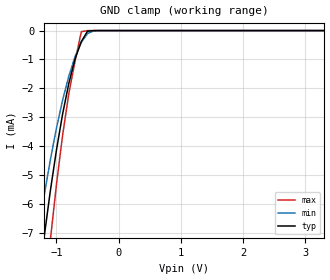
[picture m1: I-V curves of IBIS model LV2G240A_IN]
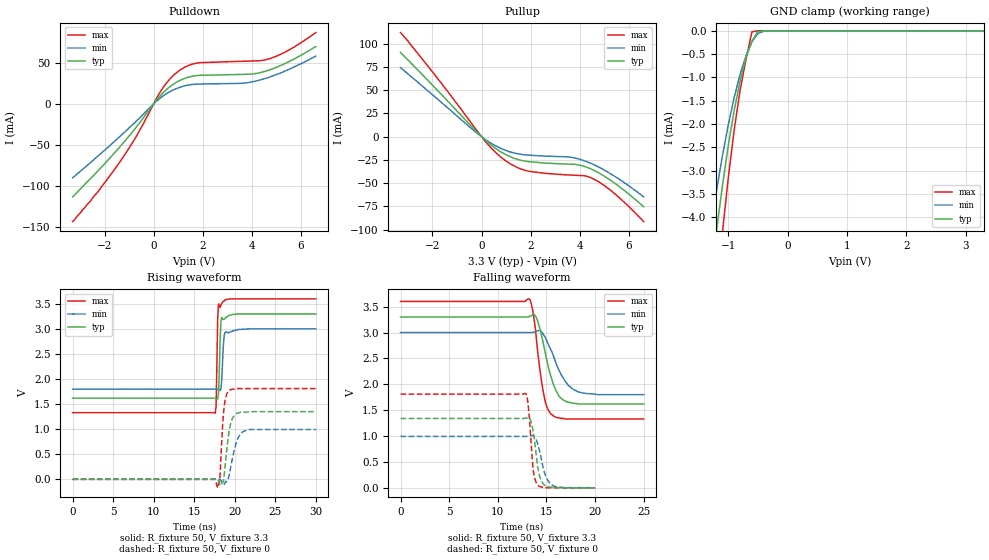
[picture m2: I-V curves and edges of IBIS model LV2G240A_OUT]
|/_/_/_/_/_/_/_/_/_/_/_/_/_/_/_/_/_/_/_/_/_/_/_/_/_/_/_/_/_/_/_/_/_/_/_/_/_/
|   Renesas Electronics Corp.
|   Multi Purpose Semiconductor Digital IC Design Group
|   IBIS Model of HD74LV2G240A
|   3.3V Dual Bus Buffer Inverted with 3-state Outputs,
|   SSOP-8(8pin) Package
|   History
|   V1.0   April   1, 2003   : First release.
|/_/_/_/_/_/_/_/_/_/_/_/_/_/_/_/_/_/_/_/_/_/_/_/_/_/_/_/_/_/_/_/_/_/_/_/_/_/
[IBIS Ver]   2.1
[Comment Char]  |_char
[File name]   l2g240s3.ibs
[File Rev]   1.1
[Date]   April 1, 2003
[Source]   Data created from SPICE simulations at
|   Renesas Electronics Corp.
[Notes]   RLC value of the Package is determined by assuming typical
|   conditions.
[Disclaimer]   This information is for modeling purposes only, and is not
|   guaranteed.
[Copyright]   Copyright 2003, Renesas Electronics Corp.,
|   All Rights Reserved.
|   Component  HD74LV2G240A
[Component]   HD74LV2G240A
[Manufacturer]  Renesas Electronics Corp.
[Package]
|   typ   min   max
R_pkg   0.099   0.095   0.102
L_pkg   1.740nH   1.680nH   1.790nH
C_pkg   0.140pF   0.140pF   0.150pF
[Pin]   signal_name   model_name   R_pin   L_pin   C_pin
1   G1   LV2G240A_IN   0.102   1.780nH   0.140pF
2   A1   LV2G240A_IN   0.097   1.710nH   0.150pF
3   Y2   LV2G240A_OUT   0.095   1.680nH   0.150pF
4   GND   GND   0.102   1.790nH   0.140pF
5   A2   LV2G240A_IN   0.101   1.790nH   0.140pF
6   Y1   LV2G240A_OUT   0.097   1.710nH   0.150pF
7   G2   LV2G240A_IN   0.097   1.710nH   0.150pF
8   VCC   POWER   0.102   1.790nH   0.140pF
| Models and submodels in the file (2): LV2G240A_IN (Input), LV2G240A_OUT (3-state)
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|   Model  LV2G240A_IN
[Model]   LV2G240A_IN
Model_type  Input
Vinl = 0.99V
Vinh = 2.31V
| variable   typ   min   max
C_comp   2.85pF   2.75pF   2.95pF
| variable   typ   min   max
[Temperature range]   25   85   -40
| variable   typ   min   max
[Voltage range]   3.3V   3.0V   3.6V
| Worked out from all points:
|   GND clamp passes 1 mA (typ) near -0.70 V on its own axis
[GND Clamp]
|   Voltage   I(typ)   I(min)   I(max)
-3.3V     -64mA      -52mA      -81.2mA
-1.3V     -8.95mA    -7.12mA    -11.9mA
-1.2V     -7.19mA    -5.75mA    -9.48mA
-1.1V     -5.58mA    -4.5mA     -7.3mA
-1V       -4.14mA    -3.38mA    -5.33mA
-900mV    -2.88mA    -2.4mA     -3.61mA
-800mV    -1.82mA    -1.57mA    -2.17mA
-700mV    -976uA     -897uA     -1.05mA
-600mV    -380uA     -405uA     -38.6uA
-500mV    -22.3uA    -104uA     -465nA
-400mV    -445nA     -10.5uA    -2.66nA
3.3V      6.7pA      30.3pA     6.6pA
|   Model  LV2G240A_OUT
[Model]   LV2G240A_OUT
Model_type  3-state
Polarity   Inverting
Enable   Active-Low
Vmeas = 1.65V
| variable   typ   min   max
C_comp   7.35pF   7.25pF   7.45pF
| variable   typ   min   max
[Temperature range]   25   85   -40
| variable   typ   min   max
[Voltage range]   3.3V   3.0V   3.6V
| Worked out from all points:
|   slope of the pulldown table from 0 to 0.495 V, typ, clamps not added: 29.9 ohm
|   slope of the pullup table from 0 to 0.495 V, typ, clamps not added: 44.6 ohm
|   GND clamp passes 1 mA (typ) near -0.78 V on its own axis
|   rising waveform, R_fixture 50, V_fixture 3.3: 20-80 % time 196ps typ, 230ps min, 153ps max; typ from 1.62 V to 3.3 V
|   rising waveform, R_fixture 50, V_fixture 0: 20-80 % time 635ps typ, 880ps min, 421ps max; typ from 0 V to 1.35 V
|   falling waveform, R_fixture 50, V_fixture 3.3: 20-80 % time 1.34ns typ, 1.77ns min, 936ps max; typ from 3.3 V to 1.62 V
|   falling waveform, R_fixture 50, V_fixture 0: 20-80 % time 600ps typ, 806ps min, 435ps max; typ from 1.34 V to 0 V
[Pullup]
|   Voltage   I(typ)   I(min)   I(max)
-3.3V     90.6mA     74.3mA     112mA
-1.7V     47.2mA     38.4mA     59.7mA
-100mV    2.6mA      2.04mA     3.43mA
300mV     -7.12mA    -5.53mA    -9.49mA
800mV     -16.5mA    -12.7mA    -22.2mA
1.2V      -21.8mA    -16.6mA    -29.6mA
1.8V      -26.3mA    -19.5mA    -36.3mA
3.6V      -29.5mA    -21.9mA    -41.1mA
4.2V      -32mA      -26mA      -42mA
4.5V      -35.2mA    -29.2mA    -44.7mA
5.4V      -49.6mA    -42.2mA    -60.8mA
6.6V      -75.3mA    -64.7mA    -91.2mA
[Pulldown]
|   Voltage   I(typ)   I(min)   I(max)
-3.3V     -113mA     -89.9mA    -143mA
-2.3V     -82.4mA    -64.3mA    -108mA
-1.4V     -53.1mA    -40.4mA    -71.6mA
-700mV    -28.1mA    -20.8mA    -39.3mA
300mV     10.8mA     7.71mA     15.9mA
600mV     19.3mA     13.7mA     28.1mA
1V        27.3mA     19.4mA     39.4mA
1.8V      34.4mA     24mA       49.6mA
3.7V      35.8mA     25.2mA     51.7mA
4.7V      41mA       32.3mA     54.6mA
5.5V      51.1mA     41.7mA     65.2mA
6.6V      69.5mA     57.9mA     86.5mA
[GND Clamp]
|   Voltage   I(typ)   I(min)   I(max)
-3.3V     -38.9mA    -31.6mA    -49.2mA
-1.3V     -5.4mA     -4.31mA    -7.13mA
-1.2V     -4.33mA    -3.47mA    -5.69mA
-1.1V     -3.36mA    -2.71mA    -4.37mA
-1V       -2.48mA    -2.03mA    -3.18mA
-900mV    -1.72mA    -1.44mA    -2.14mA
-800mV    -1.08mA    -936uA     -1.28mA
-700mV    -575uA     -533uA     -610uA
-600mV    -219uA     -237uA     -20.5uA
-500mV    -12.9uA    -58.6uA    -245nA
-400mV    -248nA     -6.13uA    -1.4nA
3.3V      3.42pA     32.9pA     3.3pA
[Ramp]
| variable   typ   min   max
dV/dt_r   0.805/630.9p   0.597/881.2p   1.087/420.5p
dV/dt_f   1.010/1.348n   0.719/1.771n   1.362/935.7p
R_load = 50ohms
[Rising Waveform]
R_fixture = 50
V_fixture = 3.3
V_fixture_min = 3.0
V_fixture_max = 3.6
C_fixture = 0p
|   Time   V(typ)   V(min)   V(max)
0s        1.62V      1.8V       1.33V
17.6ns    1.62V      1.8V       1.32V
17.7ns    1.62V      1.8V       1.45V
17.9ns    1.6V       1.8V       3.21V
18ns      1.72V      1.8V       3.5V
18.2ns    2.78V      1.77V      3.43V
18.4ns    3.23V      1.99V      3.51V
18.7ns    3.19V      2.87V      3.56V
18.9ns    3.23V      2.94V      3.58V
30ns      3.3V       3V         3.6V
[Rising Waveform]
R_fixture = 50
V_fixture = 0
C_fixture = 0p
|   Time   V(typ)   V(min)   V(max)
0s        -328nV     137nV      -29.9nV
17.6ns    -39.8uV    -48.4uV    1.65mV
17.9ns    -3.17mV    178uV      -170mV
18.2ns    -125mV     1.79mV     94.8mV
18.5ns    -60mV      -81mV      1.05V
18.7ns    79.1mV     -98.8mV    1.45V
19.3ns    947mV      72.2mV     1.77V
20.2ns    1.31V      736mV      1.81V
21.2ns    1.34V      965mV      1.81V
30ns      1.35V      994mV      1.81V
[Falling Waveform]
R_fixture = 50
V_fixture = 3.3
V_fixture_min = 3.0
V_fixture_max = 3.6
C_fixture = 0p
|   Time   V(typ)   V(min)   V(max)
0s        3.3V       3V         3.6V
13.2ns    3.31V      3V         3.65V
13.6ns    3.34V      3V         3.42V
14.1ns    3.22V      3.03V      2.63V
14.5ns    2.94V      3.01V      2.05V
14.9ns    2.59V      2.9V       1.65V
15.5ns    2.13V      2.65V      1.42V
16.5ns    1.73V      2.19V      1.34V
18.3ns    1.62V      1.85V      1.33V
25ns      1.62V      1.8V       1.33V
[Falling Waveform]
R_fixture = 50
V_fixture = 0
C_fixture = 0p
|   Time   V(typ)   V(min)   V(max)
0s        1.34V      994mV      1.81V
12.9ns    1.35V      994mV      1.82V
13.2ns    1.36V      996mV      1.45V
13.6ns    1.13V      1.01V      414mV
13.8ns    879mV      981mV      183mV
14.1ns    408mV      850mV      54.7mV
14.6ns    98mV       441mV      12.3mV
15ns      29.5mV     193mV      5.13mV
15.5ns    10.6mV     65.9mV     1.61mV
20ns      439nV      -908nV     409nV
